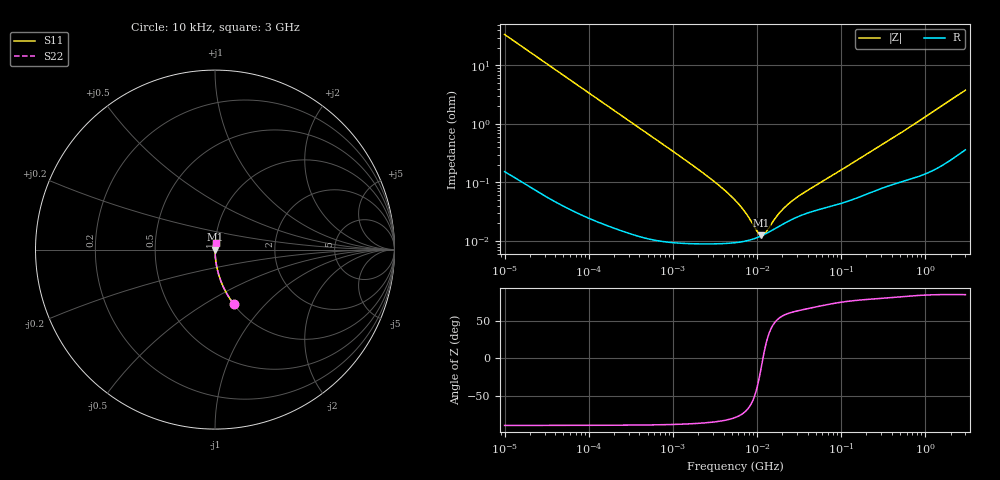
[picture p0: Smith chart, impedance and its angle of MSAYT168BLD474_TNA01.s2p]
! MSAYT168BLD474_TNA01  S-PARAMETER MODEL  ( Standard Model )
! Model Generated by TAIYO YUDEN Corporation (http://www.ty-top.com)
! Version 1.0
! TAIYO YUDEN Control No. 220601
! Copyright(c) 2013 TAIYO YUDEN CO.,LTD. All Rights Reserved.
! Product Description (link to TY-COMPAS)
! https://ds.yuden.co.jp/TYCOMPAS/or/detail?pn=MSAYT168BLD474KTNA01&u=M
! Products Name : Multilayer Ceramic Capacitors
! Characteristics :
!  Capacitance : 0.47 [uF] , Rated Voltage : 25 [V] , TCC : X5R
!  Case Size : 1.6 x 0.8 / 0.063 x 0.031 [mm/inch] , Thickness : 0.8 / 0.031 [mm/inch]
!  (Conditions: Temperature = 25 [degC] , DC Bias Voltage = 0 [V])
! External Node Assignments :
!  1  o---| |---o  2
! GND o---------o GND
! Frequency Range : 10kHz  -  3GHz  [ 401 STEP ]
# MHZ S RI R 50
! Freq[MHz].  S11 Real  S11 Imag  S21 Real  S21 Imag  S12 Real  S12 Imag  S22 Real  S22 Imag
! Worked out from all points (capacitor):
!   401 points, 10 kHz to 3 GHz, reference 50 ohm
!   read as one part in series: C = 468 nF near 10.65 kHz
!   lowest |Z| = 12.4 mohm at 11.31 MHz (marker M1)
!   series resonance near 11.78 MHz, so ESL is about 390 pH
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0.01  0.1044 -0.3035  0.8956 0.3035  0.8956 0.3035  0.1044 -0.3035
0.015549  0.0465 -0.2082  0.9535 0.2082  0.9535 0.2082  0.0465 -0.2082
0.026575  0.0168 -0.1259  0.9832 0.1259  0.9832 0.1259  0.0168 -0.1259
0.045421  0.00602 -0.0746  0.994 0.0746  0.994 0.0746  0.00602 -0.0746
0.082683  0.00198 -0.0412  0.998 0.0412  0.998 0.0412  0.00198 -0.0412
0.199902  0.000458 -0.0171  0.9995 0.0171  0.9995 0.0171  0.000458 -0.0171
0.683653  0.000125 -0.00501  0.9999 0.00501  0.9999 0.00501  0.000125 -0.00501
2.737278  9.01e-05 -0.00119  0.9999 0.00119  0.9999 0.00119  9.01e-05 -0.00119
3.996065  9.05e-05 -0.000761  0.9999 0.000761  0.9999 0.000761  9.05e-05 -0.000761
5.477226  9.32e-05 -0.000491  0.9999 0.000491  0.9999 0.000491  9.32e-05 -0.000491
7.274378  9.92e-05 -0.00029  0.9999 0.00029  0.9999 0.00029  9.92e-05 -0.00029
10.29003  0.000115 -7.71e-05  0.9999 7.71e-05  0.9999 7.71e-05  0.000115 -7.71e-05
11.31085  0.000122 -2.29e-05  0.9999 2.29e-05  0.9999 2.29e-05  0.000122 -2.29e-05
12.04705  0.000127 1.25e-05  0.9999 -1.25e-05  0.9999 -1.25e-05  0.000127 1.25e-05
12.83117  0.000133 4.74e-05  0.9999 -4.74e-05  0.9999 -4.74e-05  0.000133 4.74e-05
17.04125  0.000167 0.0002  0.9998 -0.0002  0.9998 -0.0002  0.000167 0.0002
21.93027  0.000205 0.000331  0.9998 -0.000331  0.9998 -0.000331  0.000205 0.000331
29.12589  0.000251 0.00048  0.9997 -0.00048  0.9997 -0.00048  0.000251 0.00048
45.28751  0.000318 0.000752  0.9997 -0.000752  0.9997 -0.000752  0.000318 0.000752
374.4521  0.000907 0.00521  0.9991 -0.00521  0.9991 -0.00521  0.000907 0.00521
2816.668  0.00462 0.0352  0.9954 -0.0352  0.9954 -0.0352  0.00462 0.0352
3000  0.00499 0.0373  0.995 -0.0373  0.995 -0.0373  0.00499 0.0373
